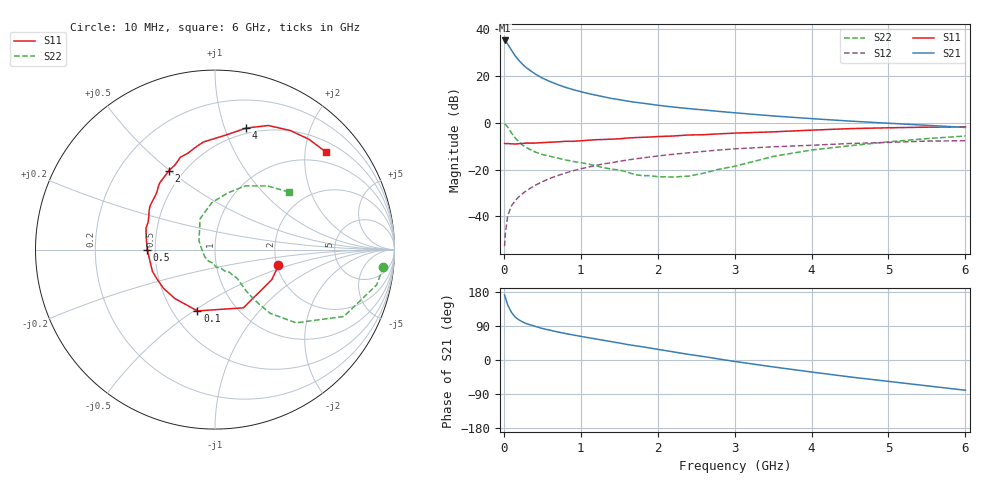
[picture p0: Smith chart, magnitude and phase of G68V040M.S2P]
! SIEMENS Small Signal Semiconductors
! BFG193
! Si NPN RF Bipolar Junction Transistor in SOT223
! VCE = 8 V  IC = 40 mA
! Common Emitter S-Parameters:  August  1996
# GHz  S  MA  R  50
!  f  S11  S21  S12  S22
! GHz  MAG  ANG  MAG  ANG  MAG  ANG  MAG  ANG
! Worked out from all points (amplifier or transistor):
!   36 points, 10 MHz to 6 GHz, reference 50 ohm
!   highest |S21| = 35.3 dB at 10 MHz (marker M1)
!   |S21| within 3 dB of that: start of sweep to 77.88 MHz
!   unconditionally stable (mu >= 1): 539.5 MHz to 2.369 GHz
!   at 250 MHz: K = 0.87, MSG = 27.5 dB, |S12| = -30.1 dB
!   at 1.4 GHz: K = 1.05, MAG = 12.4 dB, |S12| = -17.0 dB
!   at 6 GHz: K = 0.89, MSG = 2.8 dB, |S12| = -7.6 dB
!   S11 on the Smith chart (normalised r, x): 10 MHz: 2.04, -0.41; 100 MHz: 0.66, -0.52; 500 MHz: 0.45, -0.00; 2 GHz: 0.42, +0.50; 4 GHz: 0.45, +1.18; 6 GHz: 0.73, +2.47
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0.01  0.3645 -14.0  57.88 171.4  0.0023 86.4  0.9425 -5.9
0.02  0.3579 -28.0  56.22 164.7  0.0044 79.1  0.9217 -12.3
0.05  0.3609 -64.0  48.65 145.2  0.0103 71.3  0.8091 -27.4
0.1  0.3555 -106.0  35.76 125.5  0.0169 65.5  0.6086 -42.1
0.15  0.3526 -129.3  26.74 112.7  0.0219 64.0  0.47 -49.1
0.2  0.3592 -143.1  21.27 105.5  0.0267 65.2  0.3883 -51.1
0.25  0.3628 -153.7  17.44 99.8  0.0313 65.5  0.328 -52.3
0.3  0.3692 -160.9  14.8 95.4  0.0359 66.5  0.2924 -52.9
0.4  0.3686 -171.7  11.3 89.2  0.0454 66.9  0.2405 -52.7
0.5  0.3776 -179.8  9.092 83.2  0.0551 67.1  0.2104 -52.3
0.6  0.3841 173.2  7.652 78.6  0.0649 66.1  0.1924 -53.0
0.8  0.4026 162.6  5.755 69.9  0.0841 63.1  0.1612 -56.3
1.1  0.4252 149.9  4.23 58.9  0.1134 58.5  0.1315 -65.4
1.6  0.472 132.0  2.928 41.1  0.1599 48.0  0.0893 -90.4
2  0.5088 120.3  2.383 28.2  0.1951 39.3  0.0705 -131.4
2.2  0.5228 115.0  2.178 21.6  0.2128 34.8  0.0694 -149.2
2.8  0.5817 100.5  1.756 2.5  0.2626 20.9  0.1021 151.2
3.5  0.6419 84.4  1.405 -18.2  0.3075 3.9  0.191 115.7
4  0.6984 75.7  1.231 -31.7  0.3314 -5.8  0.2626 93.8
4.5  0.7523 66.8  1.09 -44.7  0.3619 -15.9  0.3239 77.3
5.5  0.8074 49.6  0.885 -68.1  0.4077 -39.1  0.4599 50.5
6  0.8233 41.3  0.798 -79.8  0.4146 -52.5  0.5227 37.8
